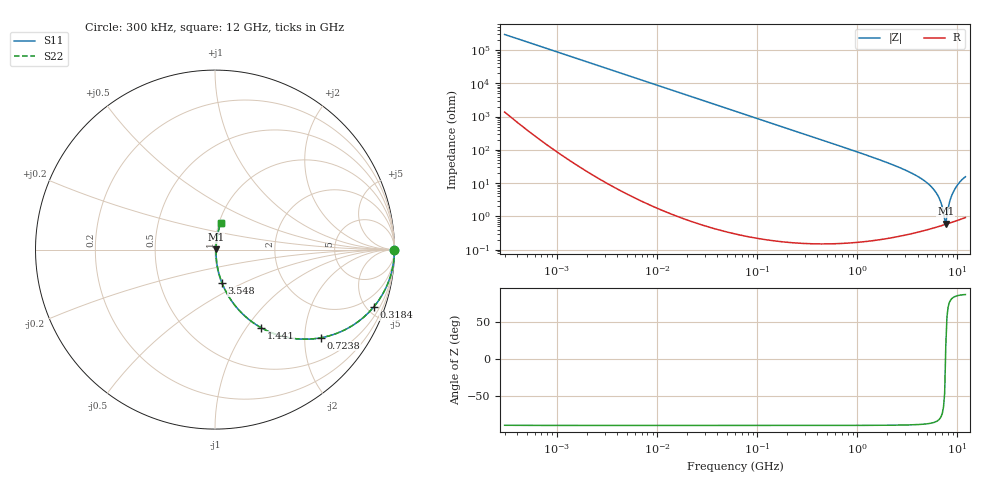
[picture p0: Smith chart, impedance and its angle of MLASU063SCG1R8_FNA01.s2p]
! MLASU063SCG1R8_FNA01  S-PARAMETER MODEL  ( Standard Model )
! Model Generated by TAIYO YUDEN Corporation (http://www.ty-top.com)
! Version 1.0
! TAIYO YUDEN Control No. 240819
! Copyright(c) 2024 TAIYO YUDEN CO.,LTD. All Rights Reserved.
! Product Description (link to TY-COMPAS)
! https://ds.yuden.co.jp/TYCOMPAS/or/detail?pn=MLASU063SCG1R8CFNA01&u=M
! Products Name : Multilayer Ceramic Capacitors
! Characteristics :
!  Capacitance : 1.8 [pF] , Rated Voltage : 50 [V] , TCC : CG / C0G
!  Case Size : 0.6 x 0.3 / 0.024 x 0.012 [mm/inch] , Thickness : 0.3 / 0.012 [mm/inch]
!  (Conditions: Temperature = 25 [degC] , DC Bias Voltage = 0 [V])
! External Node Assignments :
!  1  o---| |---o  2
! GND o---------o GND
! Frequency Range : 0.3MHz  -  12000MHz  [ 401 STEP ]
# MHZ S RI R 50
! Freq[MHz].  S11 Real  S11 Imag  S21 Real  S21 Imag  S12 Real  S12 Imag  S22 Real  S22 Imag
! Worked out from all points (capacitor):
!   401 points, 300 kHz to 12 GHz, reference 50 ohm
!   read as one part in series: C = 1.81 pF near 316.3 kHz
!   lowest |Z| = 608 mohm at 7.649 GHz (marker M1)
!   series resonance near 7.601 GHz, so ESL is about 240 pH
!   S11 on the Smith chart (normalised r, x): 300 kHz: open; 318.4 MHz: 1.00, -5.52; 723.8 MHz: 1.00, -2.41; 1.441 GHz: 1.00, -1.18; 3.548 GHz: 1.01, -0.39; 12 GHz: 1.02, +0.31
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0.3  1 -0.000341  1.7e-06 0.000341  1.7e-06 0.000341  1 -0.000341
1.769972  1 -0.00201  5.17e-06 0.00201  5.17e-06 0.00201  1 -0.00201
10.44266  0.9999 -0.0119  0.000143 0.0119  0.000143 0.0119  0.9999 -0.0119
60  0.9954 -0.0679  0.00464 0.0679  0.00464 0.0679  0.9954 -0.0679
143.8206  0.9739 -0.1592  0.0261 0.1592  0.0261 0.1592  0.9739 -0.1592
318.4019  0.8838 -0.3202  0.1162 0.3202  0.1162 0.3202  0.8838 -0.3202
353.9943  0.8601 -0.3466  0.1399 0.3466  0.1399 0.3466  0.8601 -0.3466
723.8279  0.5921 -0.4908  0.4079 0.4908  0.4079 0.4908  0.5921 -0.4908
1441.349  0.2582 -0.436  0.7418 0.436  0.7418 0.436  0.2582 -0.436
2088.533  0.1334 -0.3372  0.8666 0.3372  0.8666 0.3372  0.1334 -0.3372
3547.679  0.0392 -0.1864  0.9608 0.1864  0.9608 0.1864  0.0392 -0.1864
4747.894  0.0164 -0.1115  0.9836 0.1115  0.9836 0.1115  0.0164 -0.1115
5868.704  0.00824 -0.0607  0.9918 0.0607  0.9918 0.0607  0.00824 -0.0607
6524.734  0.00628 -0.0361  0.9937 0.0361  0.9937 0.0361  0.00628 -0.0361
6879.757  0.00579 -0.0239  0.9942 0.0239  0.9942 0.0239  0.00579 -0.0239
7254.098  0.00561 -0.0118  0.9944 0.0118  0.9944 0.0118  0.00561 -0.0118
7648.807  0.00575 0.00185  0.9942 -0.00185  0.9942 -0.00185  0.00575 0.00185
7854.144  0.00598 0.00886  0.994 -0.00886  0.994 -0.00886  0.00598 0.00886
8503.825  0.0074 0.0319  0.9926 -0.0319  0.9926 -0.0319  0.0074 0.0319
9207.246  0.0102 0.0571  0.9898 -0.0571  0.9898 -0.0571  0.0102 0.0571
10511.28  0.0189 0.1038  0.9811 -0.1038  0.9811 -0.1038  0.0189 0.1038
12000  0.032 0.1489  0.968 -0.1489  0.968 -0.1489  0.032 0.1489
